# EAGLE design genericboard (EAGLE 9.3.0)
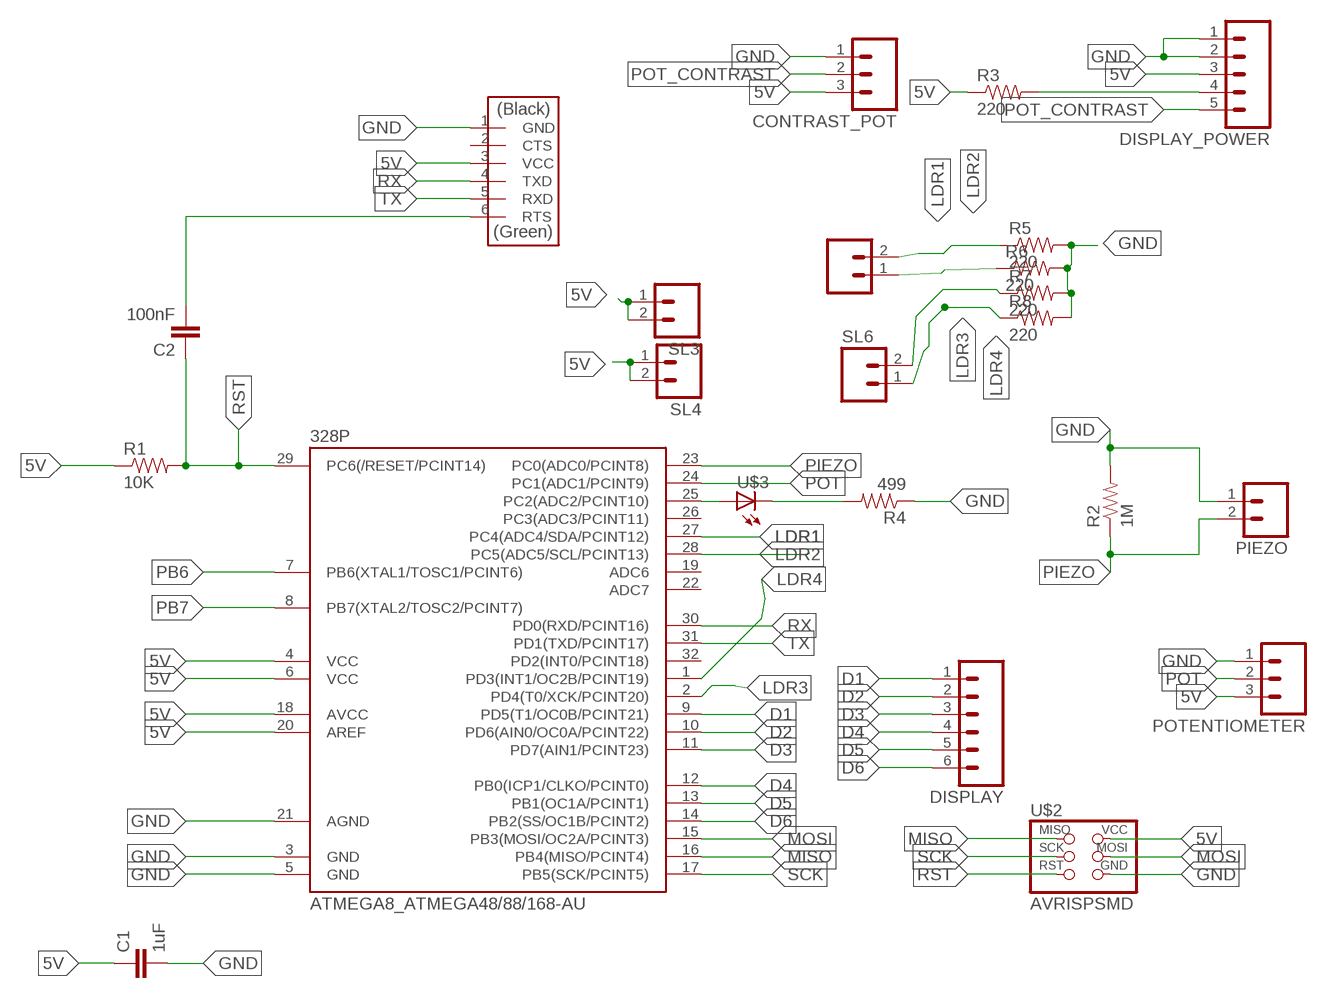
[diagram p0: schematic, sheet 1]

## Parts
328P  ATMEGA8_ATMEGA48/88/168-AU  [ATMEGA8_TQFP32-08]
C1  1uF  01_SPARKFUN_CAP1206  [01_SPARKFUN_1206]
C2  100nF  01_SPARKFUN_CAP1206  [01_SPARKFUN_1206]
CONTRAST_POT  M03  [03P]
DISPLAY  M06  [06P]
DISPLAY_POWER  M05  [05P]
FTDI  FTDI-SMD-HEADER  [1X06SMD]
PIEZO  M02  [02P]
POTENTIOMETER  M03  [03P]
R1  10K  01_SPARKFUN_RESISTOR1206  [01_SPARKFUN_1206]
R2  1M  01_SPARKFUN_RESISTOR1206  [01_SPARKFUN_1206]
R3  220  01_SPARKFUN_RESISTOR1206  [01_SPARKFUN_1206]
R4  499  01_SPARKFUN_RESISTOR1206  [01_SPARKFUN_1206]
R5  220  01_SPARKFUN_RESISTOR1206  [01_SPARKFUN_1206]
R6  220  01_SPARKFUN_RESISTOR1206  [01_SPARKFUN_1206]
R7  220  01_SPARKFUN_RESISTOR1206  [01_SPARKFUN_1206]
R8  220  01_SPARKFUN_RESISTOR1206  [01_SPARKFUN_1206]
SL3  M02  [02P]
SL4  M02  [02P]
SL5  M02  [02P]
SL6  M02  [02P]
U$2  AVRISPSMD  [2X03SMD]
U$3  01_FAB_HELLO_LED1206  [01_FAB_HELLO_1206]

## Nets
5V: 328P.4(VCC) 328P.6(VCC) 328P.18(AVCC) 328P.20(AREF) C1.1 CONTRAST_POT.3 DISPLAY_POWER.3 FTDI.3(VCC) POTENTIOMETER.3 R1.1 R3.1 SL3.1 SL3.2 SL4.1 SL4.2 U$2.2(VCC)
D1: 328P.9(PD5(T1/OC0B/PCINT21)) DISPLAY.1
D2: 328P.10(PD6(AIN0/OC0A/PCINT22)) DISPLAY.2
D3: 328P.11(PD7(AIN1/PCINT23)) DISPLAY.3
D4: 328P.12(PB0(ICP1/CLKO/PCINT0)) DISPLAY.4
D5: 328P.13(PB1(OC1A/PCINT1)) DISPLAY.5
D6: 328P.14(PB2(SS/OC1B/PCINT2)) DISPLAY.6
GND: 328P.3(GND) 328P.5(GND) 328P.21(AGND) C1.2 CONTRAST_POT.1 DISPLAY_POWER.1 DISPLAY_POWER.2 FTDI.1(GND) PIEZO.1 POTENTIOMETER.1 R2.2 R4.1 R5.2 R6.2 R7.2 R8.2 U$2.6(GND)
LDR1: 328P.27(PC4(ADC4/SDA/PCINT12)) R5.1 SL5.2
LDR2: 328P.28(PC5(ADC5/SCL/PCINT13)) R6.1 SL5.1
LDR3: 328P.2(PD4(T0/XCK/PCINT20)) R7.1 SL6.2
LDR4: 328P.1(PD3(INT1/OC2B/PCINT19)) R8.1 SL6.1
MISO: 328P.16(PB4(MISO/PCINT4)) U$2.1(MISO)
MOSI: 328P.15(PB3(MOSI/OC2A/PCINT3)) U$2.4(MOSI)
N$1: C2.2 FTDI.6(RTS)
N$2: DISPLAY_POWER.4 R3.2
N$3: 328P.25(PC2(ADC2/PCINT10)) U$3.1(A)
N$4: R4.2 U$3.2(C)
PB6: 328P.7(PB6(XTAL1/TOSC1/PCINT6))
PB7: 328P.8(PB7(XTAL2/TOSC2/PCINT7))
PIEZO: 328P.23(PC0(ADC0/PCINT8)) PIEZO.2 R2.1
POT: 328P.24(PC1(ADC1/PCINT9)) POTENTIOMETER.2
POT_CONTRAST: CONTRAST_POT.2 DISPLAY_POWER.5
RST: 328P.29(PC6(/RESET/PCINT14)) C2.1 R1.2 U$2.5(RST)
RX: 328P.30(PD0(RXD/PCINT16)) FTDI.4(TXD)
SCK: 328P.17(PB5(SCK/PCINT5)) U$2.3(SCK)
TX: 328P.31(PD1(TXD/PCINT17)) FTDI.5(RXD)
Unconnected: 328P.19(ADC6) 328P.22(ADC7) 328P.26(PC3(ADC3/PCINT11)) 328P.32(PD2(INT0/PCINT18)) FTDI.2(CTS)

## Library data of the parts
328P = satshakit_cnc:ATMEGA8_ATMEGA48/88/168
C1 C2 = satshakit_cnc:01_SPARKFUN_CAP: Capacitor
CONTRAST_POT POTENTIOMETER = con-amp-quick:M03: AMP QUICK CONNECTOR; OC_FARNELL: unknown; OC_NEWARK: unknown
DISPLAY = con-amp-quick:M06: AMP QUICK CONNECTOR; OC_FARNELL: unknown; OC_NEWARK: unknown
DISPLAY_POWER = con-amp-quick:M05: AMP QUICK CONNECTOR; OC_FARNELL: unknown; OC_NEWARK: unknown
FTDI = fab:FTDI-SMD-HEADER
PIEZO SL3-SL6 = con-amp-quick:M02: AMP QUICK CONNECTOR; OC_FARNELL: unknown; OC_NEWARK: unknown
R1-R8 = satshakit_cnc:01_SPARKFUN_RESISTOR: Resistor
U$2 = fab:AVRISP
U$3 = satshakit_cnc:01_FAB_HELLO_LED

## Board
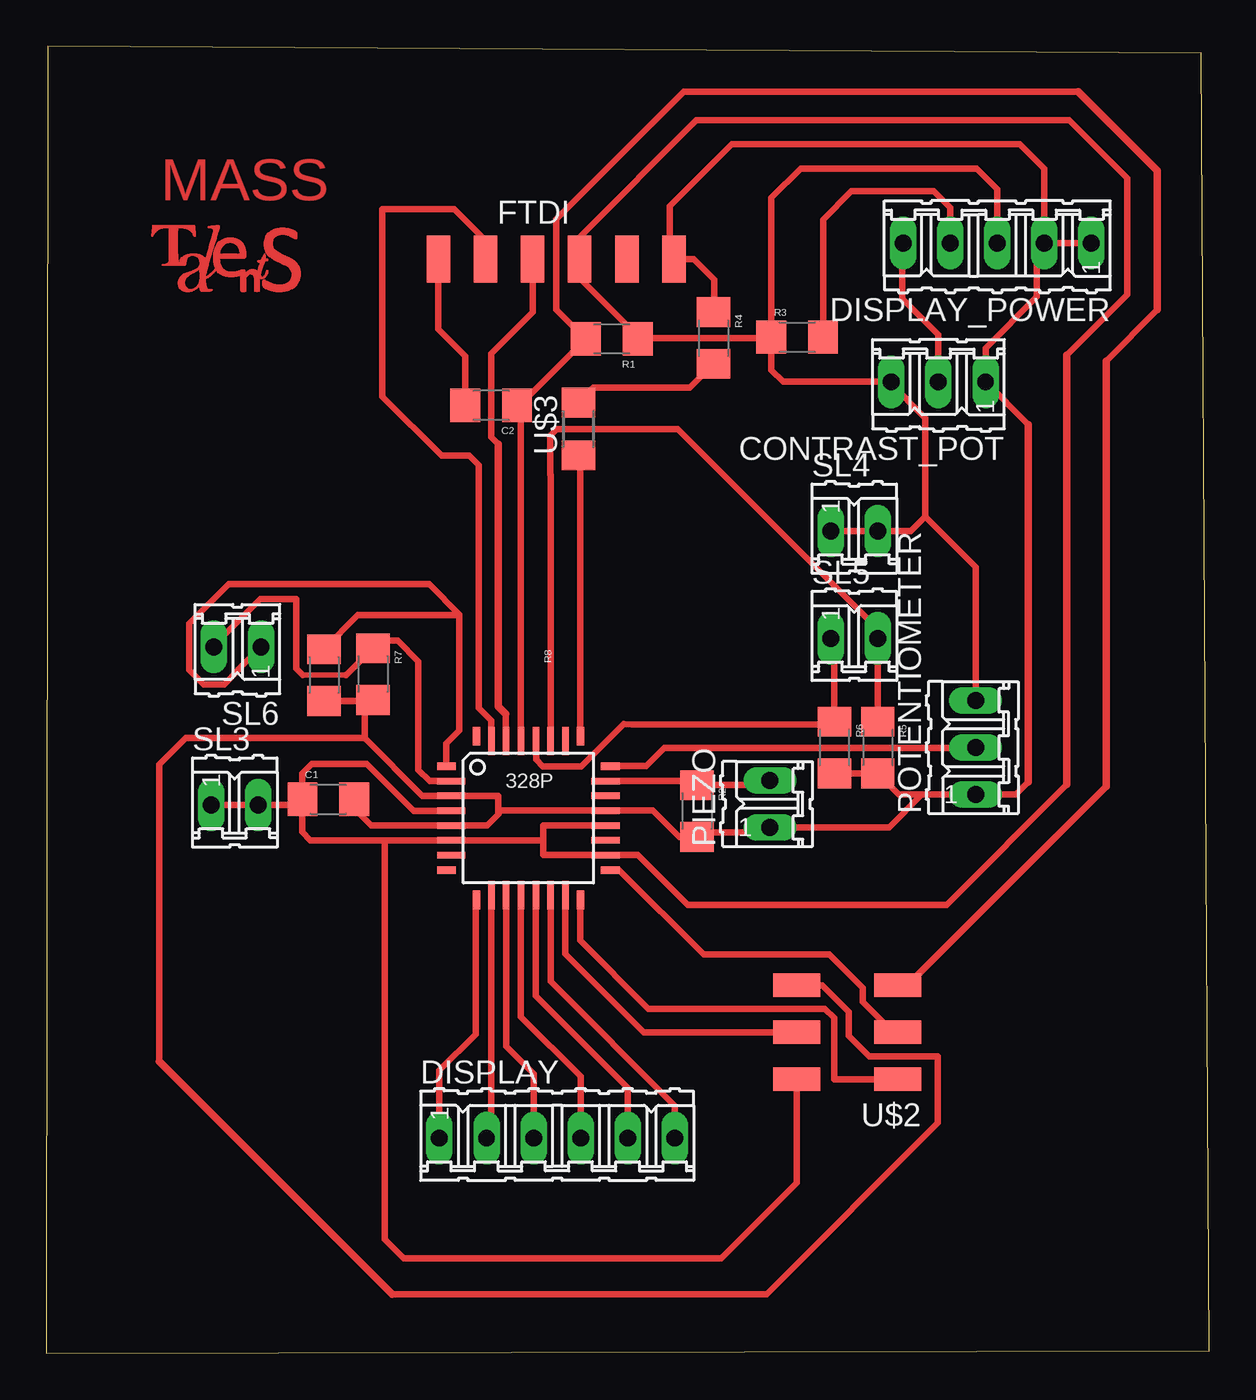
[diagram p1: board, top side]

Size 62.74 x 70.54 mm. Coordinates in mm from the lower left corner, seen from the top.
Outline: 0,0 62.74,0.13 62.31,70.16 0.08,70.54 0,0
Copper layers (1*16): Top 0.035mm / dielectric 1.5mm / Bottom 0.035mm
Design rules "default *": minimum track width 6mil, minimum drill 0.35mm, track to track 17mil, track to pad 17mil, pad to pad 17mil, via to via 17mil, smd to smd 17mil, copper to edge 40mil, drill to drill 6mil, minimum pad ring 10mil, minimum via ring 8mil, stop-mask expansion 4mil, vias tented up to drill 0mil, thermal gap 10mil

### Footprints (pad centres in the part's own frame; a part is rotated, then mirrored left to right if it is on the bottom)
ATMEGA8_TQFP32-08 = smd 1.016 x 0.406: 1 -4.42,2.8; 8 -4.42,-2.8; 17 4.42,-2.8; 24 4.42,2.8 | smd 1.524 x 0.356: 2 -4.166,2; 3 -4.166,1.2; 4 -4.166,0.4; 5 -4.166,-0.4; 6 -4.166,-1.2; 7 -4.166,-2; 18 4.166,-2; 19 4.166,-1.2; 20 4.166,-0.4; 21 4.166,0.4; 22 4.166,1.2; 23 4.166,2 | smd 0.406 x 1.016: 9 -2.8,-4.42; 16 2.8,-4.42; 25 2.8,4.42; 32 -2.8,4.42 | smd 0.356 x 1.524: 10 -2,-4.166; 11 -1.2,-4.166; 12 -0.4,-4.166; 13 0.4,-4.166; 14 1.2,-4.166; 15 2,-4.166; 26 2,4.166; 27 1.2,4.166; 28 0.4,4.166; 29 -0.4,4.166; 30 -1.2,4.166; 31 -2,4.166
01_SPARKFUN_1206 = smd 1.6 x 1.8: 1 -1.4,0; 2 1.4,0
03P = drill 0.914 long: 1 -2.54,0; 2 0,0; 3 2.54,0
06P = drill 0.914 long: 1 -6.35,0; 2 -3.81,0; 3 -1.27,0; 4 1.27,0; 5 3.81,0; 6 6.35,0
05P = drill 0.914 long: 1 -5.08,0; 2 -2.54,0; 3 0,0; 4 2.54,0; 5 5.08,0
1X06SMD = smd 2.54 x 1.27: 1 0,6.35; 2 0,3.81; 3 0,1.27; 4 0,-1.27; 5 0,-3.81; 6 0,-6.35
02P = drill 0.914 long: 1 -1.27,0; 2 1.27,0
2X03SMD = smd 2.54 x 1.27: 1 -2.54,2.54; 2 2.92,2.54; 3 -2.54,0; 4 2.92,0; 5 -2.54,-2.54; 6 2.92,-2.54
01_FAB_HELLO_1206 = smd 1.6 x 1.803: 1 -1.422,0; 2 1.422,0

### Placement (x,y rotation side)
328P  26.01,28.88 0 top
C1  15.21,29.9 0 top
C2  24,51.16 180 top
CONTRAST_POT  48.13,52.43 180 top
DISPLAY  27.56,11.61 0 top
DISPLAY_POWER  51.31,59.92 180 top
DRILEGEND  [DRILEGEND]  not placed on the board
FTDI  27.51,59.05 270 top
PIEZO  39.04,29.64 90 top
POTENTIOMETER  50.14,32.69 90 top
R1  30.51,54.74 180 top
R2  35.1,29.26 270 top
R3  40.51,54.84 0 top
R4  35.99,54.79 270 top
R5  44.86,32.69 270 top
R6  42.52,32.69 270 top
R7  17.63,36.65 270 top
R8  14.99,36.6 270 top
SL3  10.16,29.59 0 top
SL4  43.59,44.37 0 top
SL5  43.59,38.58 0 top
SL6  10.31,38.13 180 top
U$2  43.41,17.32 180 top
U$3  28.7,49.89 90 top

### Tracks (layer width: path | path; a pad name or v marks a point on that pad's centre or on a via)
5V
  Top 0.356: U$2.2 40.49,9.2 36.42,5.13 19.28,5.13 18.26,6.15 18.26,27.68 | 21.86,27.69 328P.6 | 328P.4 21.83,29.27 19.83,29.27 17.3,31.8 14.33,31.8 13.81,31.29 C1.1 | 328P.6 18.26,27.68 | 18.26,27.68 18.21,27.68 18.21,27.69 14.25,27.69 13.81,28.12 C1.1 | R3.1 39.06,54.79 31.96,54.79 R1.1 31.91,54.89 28.78,58.01 FTDI.3 28.78,60.25 35.08,66.55 55.19,66.55 58.32,63.42 58.32,57.12 55.07,53.87 | CONTRAST_POT.3 45.47,52.43 | 45.47,52.43 39.75,52.43 39.11,53.06 R3.1 | POTENTIOMETER.3 50.14,42.42 47.41,45.15 | 45.47,52.43 47.41,50.48 47.41,45.15 | DISPLAY_POWER.3 51.31,62.81 50.19,63.93 40.69,63.93 39.11,62.35 R3.1 | 55.07,30.68 48.59,24.21 34.59,24.21 31.92,26.88 328P.18 26.81,26.88 26.81,27.68 | 26.81,27.68 328P.6 | 26.81,27.68 26.81,28.48 328P.20 | SL3.1 SL3.2 13.51,29.59 C1.1 | SL4.1 SL4.2 46.63,44.37 47.41,45.15
  Top 0.406: 55.07,30.68 55.07,53.87
D1
  Top 0.356: DISPLAY.1 21.21,15.27 23.16,17.22 23.16,24.41 328P.9
D2
  Top 0.356: 23.88,11.74 DISPLAY.2 24.01,11.87 328P.10
D3
  Top 0.356: 328P.11 24.81,16.57 26.29,15.09 DISPLAY.3
D4
  Top 0.356: 328P.12 25.61,18.15 28.83,14.94 DISPLAY.4
D5
  Top 0.356: 328P.13 26.41,19.29 31.37,14.33 DISPLAY.5
D6
  Top 0.356: 328P.14 27.21,20.06 33.91,13.36 DISPLAY.6
GND
  Top 0.152: R8.2 14.27,35.2
  Top 0.356: 30.16,29.27 328P.21 | 50.27,30.02 POTENTIOMETER.1 | 328P.21 32.72,29.28 34.14,27.86 R2.2 35.36,28.12 38.78,28.12 PIEZO.1 45.47,28.37 47.24,30.15 | C1.2 16.61,29.39 17.52,28.48 328P.5 23.78,28.48 24.38,29.08 24.38,29.13 | POTENTIOMETER.1 52.3,30.15 52.98,30.84 | R4.1 36.04,56.24 36.04,57.94 34.93,59.06 FTDI.1 33.63,59.28 33.63,61.9 36.98,65.25 52.53,65.25 53.85,63.93 DISPLAY_POWER.2 | DISPLAY_POWER.2 DISPLAY_POWER.1 | 24.38,29.13 24.38,30.08 328P.3 20.29,30.07 17.17,33.2 | 328P.21 24.53,29.28 24.38,29.13 | U$2.6 41.86,19.86 43.31,18.41 43.31,17.12 44.4,16.03 48.11,16.03 48.11,12.42 38.86,3.18 18.67,3.18 | 6.1,15.75 6.1,31.78 7.52,33.2 17.17,33.2 | POTENTIOMETER.1 47.24,30.15 | DISPLAY_POWER.2 53.44,59.51 53.44,57.02 50.67,54.25 CONTRAST_POT.1 52.98,50.11 | R8.2 17.58,35.2 R7.2 17.17,34.8 17.17,33.2 | R5.2 44.64,31.29 | R6.2 R5.2 | R5.2 46,30.15 47.24,30.15
  Top 0.406: 52.98,30.84 52.98,50.11 | 18.67,3.18 6.1,15.75
LDR1
  Top 0.356: 45.42,34.09 R5.1 SL5.2 44.86,39.09 34.07,49.87 27.55,49.87 27.19,49.52 27.19,47.41 27.21,47.39 328P.27
LDR2
  Top 0.356: 328P.28 26.42,33.03 26.42,32.03 26.78,31.67 28.86,31.67 31.14,33.96 31.62,33.94 42.37,33.94 R6.1 42.52,38.38 SL5.1
LDR3
  Top 0.152: 328P.2 21.93,30.97 22.31,30.97
  Top 0.305: 13.82,36.6 16.18,36.6
  Top 0.356: SL6.2 9.04,38.2 11.53,40.69 13.48,40.69 13.48,36.95 13.82,36.6 | 328P.2 20.68,30.88 20.07,31.49 20.07,37.34 18.95,38.46 18.03,38.46 R7.1 16.18,36.6 16.15,36.6
LDR4
  Top 0.152: R8.1 14.61,38
  Top 0.356: SL6.1 10.36,36.91 10.36,36.87 9.59,36.09 8.5,36.09 7.72,36.87 7.72,39.38 9.84,41.5 20.65,41.5 22.29,39.87 | 22.29,39.87 22.29,33.6 21.59,32.9 328P.1 | R8.1 16.81,39.83 22.25,39.83 22.29,39.87
MISO
  Top 0.356: 328P.16 28.81,22.27 32.49,18.59 42.01,18.59 42.52,18.09 42.52,14.78 U$2.1
MOSI
  Top 0.356: 328P.15 28.01,21.55 32.23,17.32 U$2.4
N$1
  Top 0.356: C2.2 22.6,53.83 21.16,55.27 FTDI.6
N$2
  Top 0.356: R3.2 41.91,61.19 43.43,62.71 47.88,62.71 48.77,61.82 DISPLAY_POWER.4
N$3
  Top 0.356: 328P.25 28.81,48.36 U$3.1
N$4
  Top 0.356: U$3.2 29.51,52.12 34.72,52.12 R4.2
PIEZO
  Top 0.356: PIEZO.2 38.79,30.66 R2.1 34.88,30.88 328P.23
POT
  Top 0.356: POTENTIOMETER.2 50.11,32.66 33.35,32.66 32.38,31.69 30.44,31.69 328P.24
POT_CONTRAST
  Top 0.356: CONTRAST_POT.2 48.13,54.97 46.18,56.92 46.18,59.87 DISPLAY_POWER.5
RST
  Top 0.356: 328P.29 25.61,50.95 C2.1 25.52,51.16 R1.2 | 57.18,53.54 59.94,56.31 | 55.68,68.1 34.39,68.1 27.51,61.21 27.51,56.33 R1.2 | 28.45,55.39 R1.2
  Top 0.381: 57.18,30.58 46.46,19.86 U$2.5
  Top 0.406: 57.18,30.58 57.18,53.54 | 59.94,56.31 59.94,63.83 55.68,68.1
RX
  Top 0.356: 24.38,49.08 24,49.45 24,53.95 26.24,56.19 FTDI.4 | 24.8,34.5 24.8,34.46 24.8,33.06 328P.30
  Top 0.406: 24.38,49.08 24.38,36.62 24.38,36.63 24.38,34.91 24.8,34.5
SCK
  Top 0.356: 328P.17 30.89,26.08 35.46,21.51 42.24,21.51 44.04,19.71 44.04,18.97 45.57,17.45 45.57,17.32 | 45.31,17.32 45.57,17.32 | 45.57,17.32 U$2.3
TX
  Top 0.356: 328P.31 24.01,34.14 23.32,34.82 23.32,47.92 22.81,48.44 21.34,48.44 18.14,51.64 18.14,61.75 22,61.75 23.52,60.22 23.52,59.23 FTDI.5
(copper drawn outside any net)
  shapes: Top area x759

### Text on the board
Top: MASS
